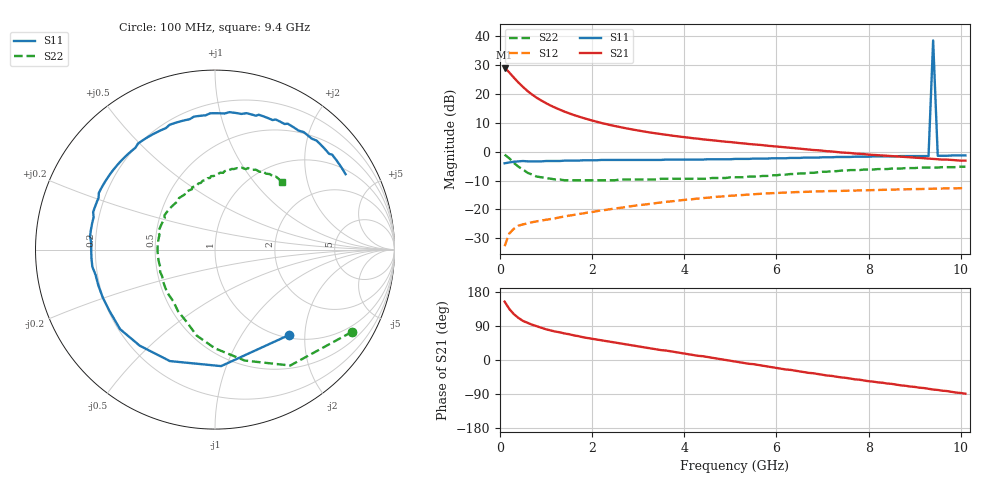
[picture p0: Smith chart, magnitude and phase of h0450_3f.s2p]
!HBFP-0450
!S and NOISE PARAMETERS at Vce=3V  Ic=20mA.  LAST UPDATED  09-04-98
# GHZ S MA R  50
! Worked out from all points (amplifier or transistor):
!   101 points, 100 MHz to 10.1 GHz, reference 50 ohm
!   highest |S21| = 29.2 dB at 100 MHz (marker M1)
!   |S21| within 3 dB of that: start of sweep to 275 MHz
!   unconditionally stable (mu >= 1): 2.454 GHz to 9.306 GHz; 9.495 GHz to end of sweep
!   at 1.7 GHz: K = 0.89, MSG = 16.9 dB, |S12| = -21.6 dB
!   at 5.1 GHz: K = 1.10, MAG = 7.3 dB, |S12| = -15.2 dB
!   at 10.1 GHz: K = 1.05, MAG = 3.4 dB, |S12| = -12.7 dB
!   lowest NFmin = 1.31 dB at 1.8 GHz
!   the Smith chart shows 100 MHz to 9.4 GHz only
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0.1  0.63 -49.0  28.7 154.0  0.023 68.0  0.89 -31.0
0.2  0.65 -87.0  23.71 135.0  0.038 53.0  0.77 -57.0
0.3  0.67 -112.0  19.3 121.0  0.046 44.0  0.64 -75.0
0.4  0.68 -128.0  15.83 111.0  0.052 38.0  0.55 -90.0
0.5  0.69 -140.0  13.26 103.0  0.055 35.0  0.49 -102.0
0.6  0.68 -150.0  11.23 98.0  0.057 33.0  0.43 -112.0
0.7  0.68 -157.0  9.76 93.0  0.06 32.0  0.4 -121.0
0.8  0.68 -163.0  8.6 89.0  0.062 31.0  0.37 -129.0
1  0.69 -172.0  6.94 81.0  0.066 31.0  0.35 -142.0
1.2  0.69 -180.0  5.79 75.0  0.07 31.0  0.33 -153.0
1.4  0.7 174.0  4.96 70.0  0.075 31.0  0.32 -162.0
1.8  0.71 163.0  3.86 60.0  0.085 30.0  0.32 -176.0
2.2  0.72 154.0  3.15 52.0  0.096 28.0  0.32 172.0
2.5  0.72 148.0  2.78 46.0  0.104 27.0  0.32 165.0
3.5  0.72 128.0  2.02 26.0  0.132 19.0  0.34 146.0
5.1  0.75 99.0  1.44 -4.0  0.174 0.0  0.36 115.0
6.8  0.79 68.0  1.07 -35.0  0.204 -23.0  0.43 84.0
8.5  0.83 42.0  0.84 -63.0  0.22 -45.0  0.51 59.0
9.3  0.84 30.0  0.76 -76.0  0.227 -56.0  0.53 47.0
9.4  85 29.0  0.75 -78.0  0.228 -57.0  0.53 45.0
9.5  0.85 27.0  0.74 -79.0  0.229 -59.0  0.53 44.0
10.1  0.86 18.0  0.7 -89.0  0.233 -68.0  0.55 34.0
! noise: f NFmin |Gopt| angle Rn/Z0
1.8  1.31  0.47  -167  0
2  1.36  0.49  -164  0
2.5  1.49  0.52  -152  0
3.5  1.75  0.59  -132  0
4  1.87  0.63  -121  0
5  2.13  0.67  -102  1
5.5  2.26  0.7  -92  1
7  2.64  0.77  -64  2
8  2.9  0.81  -47  3
10  3.41  0.83  -18  5
